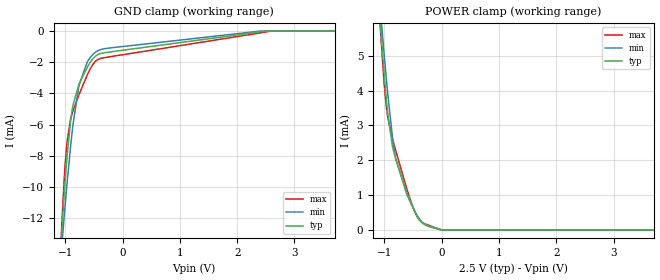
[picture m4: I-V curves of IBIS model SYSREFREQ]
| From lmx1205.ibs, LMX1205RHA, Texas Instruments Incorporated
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|   Model SYSREFREQ
[Model]   SYSREFREQ
Model_type   Input
Vinl = 0.4
Vinh = 1.4
|   typ   min   max
C_comp   0.373pF   0.304pF   0.455pF
[Voltage Range]   2.5   2.4   2.6
[Temperature Range]   27   105   -40
[Power Clamp Reference]   2.5   2.4   2.6
[GND Clamp Reference]   0   0   0
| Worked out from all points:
|   POWER clamp passes 1 mA (typ) near -0.59 V on its own axis
[GND Clamp]
|   Voltage   I(typ)   I(min)   I(max)
-2.5V     -127.7mA   -96.61mA   -208.9mA
-1.127V   -16.93mA   -16.92mA   -18.39mA
-1.06V    -12.72mA   -13.73mA   -12.28mA
-1.008V   -9.834mA   -11.39mA   -8.783mA
-970mV    -8.062mA   -9.807mA   -7.128mA
-910mV    -5.855mA   -7.497mA   -5.693mA
-865mV    -4.747mA   -5.989mA   -5.102mA
-760mV    -3.39mA    -3.463mA   -4.069mA
-617.5mV  -2.323mA   -1.989mA   -2.824mA
-422.5mV  -1.494mA   -1.242mA   -1.807mA
2.592V    0A         0A         -4.228uA
5V        0A         0A         0A
[POWER Clamp]
|   Voltage   I(typ)   I(min)   I(max)
-2.5V     54.52mA    54.1mA     56.44mA
-1.367V   12.32mA    12.12mA    12.91mA
-1.008V   4.516mA    5.078mA    4.229mA
-940mV    3.29mA     3.868mA    3.215mA
-857.5mV  2.368mA    2.618mA    2.607mA
-805mV    2.043mA    2.048mA    2.288mA
-617.5mV  1.128mA    1.06mA     1.217mA
-467.5mV  516.5uA    527.1uA    514.5uA
-377.5mV  266.9uA    287.8uA    265.7uA
-242.5mV  122.4uA    111.5uA    142.7uA
12.5mV    0A         0A         0A
5V        0A         0A         0A
